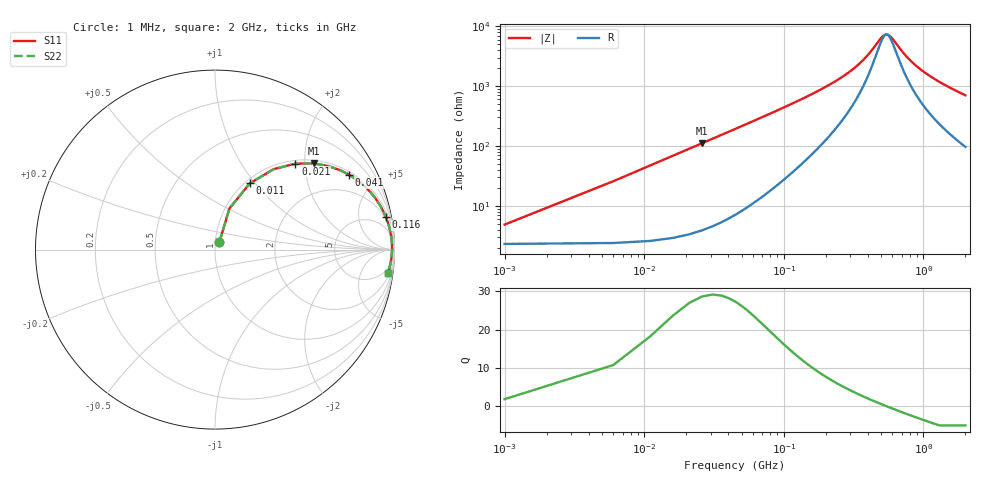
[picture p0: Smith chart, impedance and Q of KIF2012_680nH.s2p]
!version-2
!date-12.2020
!Series
# MHz S RI R 50
!Freq ReS11 ImS11 ReS21 ImS21 ReS12 ImS12 ReS22 ImS22
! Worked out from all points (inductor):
!   401 points, 1 MHz to 2 GHz, reference 50 ohm
!   read as one part in series: L = 679 nH near 11 MHz
!   highest Q = 27 at 26 MHz (marker M1), where L = 681 nH
!   self-resonance near 545.3 MHz
!   S11 on the Smith chart (normalised r, x): 1 MHz: 1.05, +0.09; 11 MHz: 1.05, +0.94; 21 MHz: 1.07, +1.79; 41 MHz: 1.13, +3.52; 116 MHz: 2, +10; 2 GHz: 3, -14
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1  0.0242 0.0407  0.9758 -0.0407  0.9758 -0.0407  0.0242 0.0407
11  0.194 0.3689  0.806 -0.3689  0.806 -0.3689  0.194 0.3689
16  0.3256 0.4479  0.6744 -0.4479  0.6744 -0.4479  0.3256 0.4479
21  0.4483 0.4791  0.5517 -0.4791  0.5517 -0.4791  0.4483 0.4791
26  0.5513 0.4802  0.4487 -0.4802  0.4487 -0.4802  0.5513 0.4802
31  0.6336 0.465  0.3664 -0.465  0.3664 -0.465  0.6336 0.465
41  0.7483 0.4165  0.2517 -0.4165  0.2517 -0.4165  0.7483 0.4165
51  0.8189 0.3663  0.1811 -0.3663  0.1811 -0.3663  0.8189 0.3663
66  0.8803 0.303  0.1197 -0.303  0.1197 -0.303  0.8803 0.303
116  0.9521 0.181  0.0479 -0.181  0.0479 -0.181  0.9521 0.181
191  0.976 0.1036  0.024 -0.1036  0.024 -0.1036  0.976 0.1036
336  0.9852 0.042  0.0148 -0.042  0.0148 -0.042  0.9852 0.042
486  0.9866 0.00961  0.0134 -0.00961  0.0134 -0.00961  0.9866 0.00961
526  0.9866 0.003  0.0134 -0.003  0.0134 -0.003  0.9866 0.003
551  0.9865 -0.000866  0.0135 0.000866  0.0135 0.000866  0.9865 -0.000866
576  0.9865 -0.00456  0.0135 0.00456  0.0135 0.00456  0.9865 -0.00456
671  0.9859 -0.0173  0.0141 0.0173  0.0141 0.0173  0.9859 -0.0173
811  0.9845 -0.0336  0.0155 0.0336  0.0155 0.0336  0.9845 -0.0336
1001  0.9821 -0.0529  0.0179 0.0529  0.0179 0.0529  0.9821 -0.0529
1336  0.9766 -0.0824  0.0234 0.0824  0.0234 0.0824  0.9766 -0.0824
1671  0.97 -0.1087  0.03 0.1087  0.03 0.1087  0.97 -0.1087
2000  0.9627 -0.1327  0.0373 0.1327  0.0373 0.1327  0.9627 -0.1327
